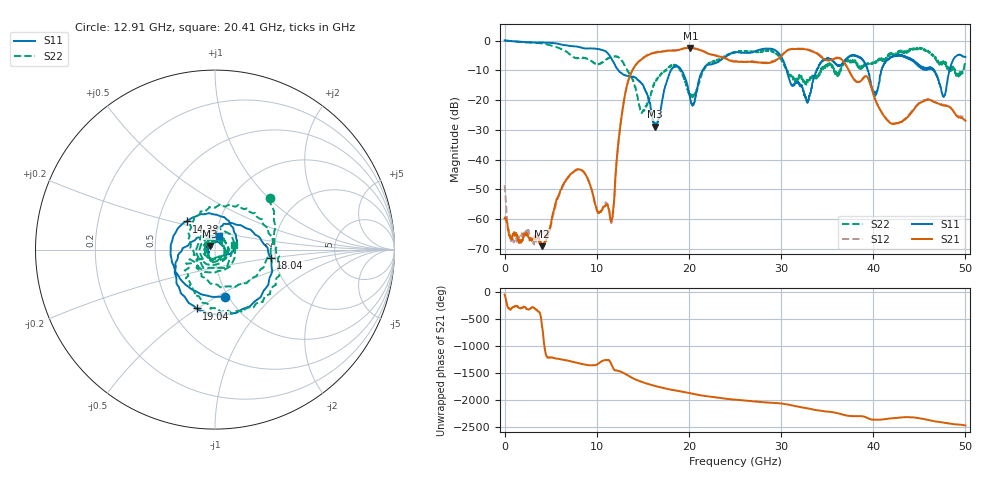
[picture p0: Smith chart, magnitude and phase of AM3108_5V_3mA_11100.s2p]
# Hz S DB R 50.0
!freq dBS11 angS11 dBS21 angS21 dBS12 angS12 dBS22 angS22
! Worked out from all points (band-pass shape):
!   1601 points, 10 MHz to 50 GHz, reference 50 ohm
!   highest |S21| = -2.47 dB at 20.16 GHz (marker M1); lowest = -69.1 dB at 4.04 GHz (marker M2)
!   |S21| within 3 dB of the highest: 15.24 GHz to 23.44 GHz (8.205 GHz wide, 42.4 % of centre); 29.93 GHz to 34.32 GHz (4.391 GHz wide, 13.7 % of centre)
!   lowest |S11| = -28.9 dB at 16.32 GHz (marker M3), VSWR 1.07, Z = 47 + j1.84 ohm
!   |S11| at or under -10 dB: 12.34 GHz to 18.04 GHz (5.709 GHz wide, 37.6 % of centre); 19.18 GHz to 21.49 GHz (2.305 GHz wide, 11.3 % of centre); 30.62 GHz to 33.85 GHz (3.229 GHz wide, 10 % of centre)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
!   |S22| runs from -24.3 to 0.0 dB; largest |S21 - S12| = 0.024
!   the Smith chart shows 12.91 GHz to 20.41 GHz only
!   S11 on the Smith chart (normalised r, x): 12.91 GHz: 0.97, -0.55; 14.38 GHz: 0.70, +0.23; 18.04 GHz: 1.89, -0.20; 19.04 GHz: 0.67, -0.50; 20.41 GHz: 1.03, +0.16
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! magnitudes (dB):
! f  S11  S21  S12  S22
! 10 MHz  0.0  -59.7  -48.6  0.0
! 853.6 MHz  -0.2  -66.1  -67.4  -0.2
! 4.04 GHz  -0.7  -69.1  -65.0  -1.0
! 8.352 GHz  -2.4  -43.6  -43.5  -5.7
! 11.6 GHz  -6.0  -60.6  -61.3  -5.6
! 12.91 GHz  -11.4  -21.0  -21.0  -7.6
! 14.38 GHz  -13.1  -7.6  -7.5  -18.5
! 16.32 GHz  -28.9  -4.1  -3.9  -14.1
! 16.69 GHz  -26.9  -3.8  -3.6  -12.6
! 18.04 GHz  -10.0  -3.4  -3.3  -8.5
! 19.04 GHz  -9.3  -3.0  -3.1  -9.6
! 20.16 GHz  -20.1  -2.5  -2.4  -18.5
! 20.41 GHz  -21.8  -2.5  -2.5  -19.1
! 21.72 GHz  -8.9  -3.8  -3.8  -9.4
! 25 GHz  -3.9  -7.1  -7.0  -4.0
! 29.25 GHz  -3.1  -7.0  -6.8  -3.9
! 33.35 GHz  -15.8  -3.6  -3.4  -12.7
! 37.91 GHz  -4.9  -13.1  -13.0  -6.5
! 40.22 GHz  -18.6  -19.8  -19.6  -7.6
! 41.69 GHz  -6.1  -27.2  -27.1  -5.2
! 47.66 GHz  -19.0  -21.9  -21.6  -7.7
! 50 GHz  -5.5  -26.9  -26.4  -6.9
